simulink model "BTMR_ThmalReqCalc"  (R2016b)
settings: Solver=FixedStepDiscrete  StartTime=0.0  StopTime=10.0  FixedStep=0.1  RelTol=1e-3  EnableMultiTasking=on
undefined symbols (not defined in the file or in its folder): BMS_cntThmStbNum_C, BTMR_cntThmalReqVal_C, BTMR_flgCoolPwrCal_C, BTMR_pChrgClntPwrLv1_C, BTMR_pChrgClntPwrLv2_C, BTMR_pChrgClntPwrLv3_C, BTMR_pChrgClntPwrLv4_C, BTMR_pChrgClntPwrLv5_C, BTMR_pChrgClntPwrLv6_C, BTMR_pCoolPwrVal_C, BTMR_pHtgACPwrReq_C, BTMR_pHtgDCPwrReq_C, BTMR_pHtgDrvPwrReq_C, BTMR_pHtgsStage1_CUR, BTMR_pHtgsStage2_CUR, BTMR_pNormClntPwrLv1_C, BTMR_pNormClntPwrLv2_C, BTMR_pNormClntPwrLv3_C, BTMR_r861BrsDrvSoc_C, BTMR_r861HtgDrvSoc_C, BTMR_r891BrsDrvSoc_C, BTMR_r891HtgDrvSoc_C, BTMR_rCoolClbFlg_C, BTMR_rFlashClbFlg_C, BTMR_rHeatClbFlg_C, BTMR_t861BrsDiffLv0Temp_C, BTMR_t861BrsDiffLv1Temp_C, BTMR_t861CoolChrgAces2Temp_C, BTMR_t861CoolChrgAces3Temp_C, BTMR_t861CoolChrgAcesTemp_C, BTMR_t861CoolChrgDiffDebTemp_C, BTMR_t861CoolChrgEndDiffTemp_C, BTMR_t861CoolChrgExitLv2Temp_C, BTMR_t861CoolChrgExitLv3Temp_C, BTMR_t861CoolChrgExitTemp_C, BTMR_t861CoolChrgIntLv0Temp_C, BTMR_t861CoolChrgIntLv1Temp_C, BTMR_t861CoolChrgIntLv2Temp_C, BTMR_t861CoolChrgIntLv3Temp_C, BTMR_t861CoolChrgIntLv4Temp_C, BTMR_t861CoolChrgIntLv5Temp_C, BTMR_t861CoolDCDebTemp_C, BTMR_t861CoolNormAcesTemp_C, BTMR_t861CoolNormDiffDebTemp_C, BTMR_t861CoolNormEndDiffTemp_C, BTMR_t861CoolNormExitLv2Temp_C, BTMR_t861CoolNormExitLv3Temp_C, BTMR_t861CoolNormExitTemp_C, BTMR_t861CoolNormIntLv0Temp_C, BTMR_t861CoolNormIntLv1Temp_C, BTMR_t861CoolNormLv2Temp_C, BTMR_t861CoolNormLv3Temp_C, BTMR_t861HtgACDiffDebTemp_C, BTMR_t861HtgACEndDiffTemp_C, BTMR_t861HtgACStartHiTemp_C, BTMR_t861HtgACStartLoTemp_C, BTMR_t861HtgACStopTemp_C, BTMR_t861HtgDCDiffDebTemp_C, BTMR_t861HtgDCEndDiffTemp_C, BTMR_t861HtgDCIntLv0Temp_C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
libraries: AIWAYS_Powertrain_BMS_lib x78, simulink x9
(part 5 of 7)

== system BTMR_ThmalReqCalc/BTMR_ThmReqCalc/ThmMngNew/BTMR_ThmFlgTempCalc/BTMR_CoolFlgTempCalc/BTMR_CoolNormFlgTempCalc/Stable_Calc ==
  source_Uint : Inport
  cntStable : Inport  Port=2
  Chart : Stateflow chart  TreatAsAtomicUnit=on
  Delay1 : Delay  DelayLength=1  InitialCondition=0
  Detect Change : simulink/Logic and Bit Operations/Detect Change  vinit=0  OutDataTypeStr=boolean
  Switch : Switch  Criteria=u2 ~= 0
  stableOut : Outport
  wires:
  source_Uint/1 -> Detect Change/1, Switch/3
  Switch/1 -> stableOut/1, Delay1/1
  Delay1/1 -> Switch/1
  Chart/1(flg_out) -> Switch/2
  cntStable/1 -> Chart/2(cntStable)
  Detect Change/1 -> Chart/1(trigger_in)

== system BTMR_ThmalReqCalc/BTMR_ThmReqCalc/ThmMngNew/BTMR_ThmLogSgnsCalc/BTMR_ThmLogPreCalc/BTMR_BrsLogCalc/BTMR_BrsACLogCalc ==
  BTMR_flgBMSStsSgns : Inport
  BTMR_flgBrsEnSgns : Inport  Port=2
  BTMR_flgBrsIntSgns : Inport  Port=3
  Bus Creator : BusCreator  Inputs=3
  Bus Selector : BusSelector  OutputSignals=BTMR_flgBMSAChrg
  Bus Selector2 : BusSelector  OutputSignals=BTMR_flgBrsEna2Temp
  Bus Selector3 : BusSelector  OutputSignals=BTMR_flgBrsIntEna2Temp
  Logical Operator1 : Logic  Operator=NOT  AllPortsSameDT=off  OutDataTypeStr=boolean
  Logical Operator{2..4,6} (4 alike) : Logic  AllPortsSameDT=off  OutDataTypeStr=boolean
  Logical Operator5 : Logic  Operator=NOT  AllPortsSameDT=off  OutDataTypeStr=boolean
  BTMR_flgBrsACLogSgns : Outport
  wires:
  Bus Selector3/1 -> Logical Operator5/1, Logical Operator3/2  "<BTMR_flgBrsIntEna2Temp>"
  Logical Operator6/1 -> Logical Operator3/1, Logical Operator4/1  "BTMR_flgBrsEna2"
  Logical Operator2/1 -> Bus Creator/2  "BTMR_flgBrsACOut"
  Logical Operator1/1 -> Logical Operator2/2
  Bus Selector/1 -> Logical Operator2/1, Logical Operator6/1  "<BTMR_flgBMSAChrg>"
  BTMR_flgBrsEnSgns/1 -> Bus Selector2/1
  BTMR_flgBrsIntSgns/1 -> Bus Selector3/1
  BTMR_flgBMSStsSgns/1 -> Bus Selector/1
  Logical Operator4/1 -> Bus Creator/3  "BTMR_flgBrsACout2"
  Bus Selector2/1 -> Logical Operator1/1, Logical Operator6/2  "<BTMR_flgBrsEna2Temp>"
  Logical Operator3/1 -> Bus Creator/1  "BTMR_flgBrsIntEna2"
  Logical Operator5/1 -> Logical Operator4/2
  Bus Creator/1 -> BTMR_flgBrsACLogSgns/1  "BTMR_flgBrsACLogSgns"

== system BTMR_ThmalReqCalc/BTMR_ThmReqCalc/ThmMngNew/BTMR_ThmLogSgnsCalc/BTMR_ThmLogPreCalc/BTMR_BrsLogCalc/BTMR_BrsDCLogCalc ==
  BTMR_flgBMSStsSgns : Inport
  BTMR_flgBrsEnSgns : Inport  Port=2
  BTMR_flgBrsIntSgns : Inport  Port=3
  Bus Creator : BusCreator  Inputs=3
  Bus Selector : BusSelector  OutputSignals=BTMR_flgBMSDChrg
  Bus Selector2 : BusSelector  OutputSignals=BTMR_flgBrsEna1Temp
  Bus Selector3 : BusSelector  OutputSignals=BTMR_flgBrsIntEna1Temp
  Logical Operator1 : Logic  Operator=NOT  AllPortsSameDT=off  OutDataTypeStr=boolean
  Logical Operator{2..4,6} (4 alike) : Logic  AllPortsSameDT=off  OutDataTypeStr=boolean
  Logical Operator5 : Logic  Operator=NOT  AllPortsSameDT=off  OutDataTypeStr=boolean
  BTMR_flgBrsDCLogSgns : Outport
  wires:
  Bus Creator/1 -> BTMR_flgBrsDCLogSgns/1  "BTMR_flgBrsDCLogSgns"
  Logical Operator5/1 -> Logical Operator4/2
  Logical Operator3/1 -> Bus Creator/1  "BTMR_flgBrsIntEna1"
  Bus Selector2/1 -> Logical Operator6/2, Logical Operator1/1  "<BTMR_flgBrsEna1Temp>"
  Logical Operator4/1 -> Bus Creator/3  "BTMR_flgBrsDCout2"
  BTMR_flgBMSStsSgns/1 -> Bus Selector/1
  BTMR_flgBrsIntSgns/1 -> Bus Selector3/1
  BTMR_flgBrsEnSgns/1 -> Bus Selector2/1
  Bus Selector/1 -> Logical Operator6/1, Logical Operator2/1  "<BTMR_flgBMSDChrg>"
  Logical Operator1/1 -> Logical Operator2/2
  Logical Operator2/1 -> Bus Creator/2  "BTMR_flgBrsDCOut"
  Logical Operator6/1 -> Logical Operator3/1, Logical Operator4/1  "BTMR_flgBrsEna1"
  Bus Selector3/1 -> Logical Operator3/2, Logical Operator5/1  "<BTMR_flgBrsIntEna1Temp>"

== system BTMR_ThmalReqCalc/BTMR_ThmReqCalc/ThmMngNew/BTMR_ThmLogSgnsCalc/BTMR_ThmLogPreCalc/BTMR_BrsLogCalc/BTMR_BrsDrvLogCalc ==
  BTMR_flgBMSStsSgns : Inport
  BTMR_flgBrsEnSgns : Inport  Port=2
  BTMR_flgBrsIntSgns : Inport  Port=3
  BTMR_flgSOCSgns : Inport  Port=4
  Bus Creator : BusCreator  Inputs=4
  Bus Selector : BusSelector  OutputSignals=BTMR_flgBMSDrv
  Bus Selector1 : BusSelector  OutputSignals=BTMR_flgBrsDrvSOC
  Bus Selector2 : BusSelector  OutputSignals=BTMR_flgBrsEna3Temp
  Bus Selector3 : BusSelector  OutputSignals=BTMR_flgBrsIntEna3Temp
  Logical Operator1 : Logic  Operator=NOT  AllPortsSameDT=off  OutDataTypeStr=boolean
  Logical Operator{2..4,6..7,9} (6 alike) : Logic  AllPortsSameDT=off  OutDataTypeStr=boolean
  Logical Operator5 : Logic  Operator=NOT  AllPortsSameDT=off  OutDataTypeStr=boolean
  Logical Operator8 : Logic  Operator=NOT  AllPortsSameDT=off  OutDataTypeStr=boolean
  BTMR_flgBrsDrvLogSgns : Outport
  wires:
  Bus Creator/1 -> BTMR_flgBrsDrvLogSgns/1  "BTMR_flgBrsDrvLogSgns"
  Logical Operator5/1 -> Logical Operator4/2
  Logical Operator7/1 -> Bus Creator/1  "BTMR_flgBrsIntEna3"
  Bus Selector2/1 -> Logical Operator1/1, Logical Operator6/2  "<BTMR_flgBrsEna3Temp>"
  Logical Operator9/1 -> Bus Creator/3  "BTMR_flgBrsDrvOut2"
  BTMR_flgBMSStsSgns/1 -> Bus Selector/1
  BTMR_flgBrsIntSgns/1 -> Bus Selector3/1
  BTMR_flgBrsEnSgns/1 -> Bus Selector2/1
  Bus Selector/1 -> Logical Operator6/1, Logical Operator2/1  "<BTMR_flgBMSDrv>"
  Logical Operator1/1 -> Logical Operator2/2
  Logical Operator6/1 -> Logical Operator9/1, Logical Operator3/1  "BTMR_flgBrsEna3"
  Bus Selector3/1 -> Logical Operator5/1, Logical Operator7/2  "<BTMR_flgBrsIntEna3Temp>"
  BTMR_flgSOCSgns/1 -> Bus Selector1/1
  Bus Selector1/1 -> Logical Operator3/2, Logical Operator8/1  "<BTMR_flgBrsDrvSOC>"
  Logical Operator3/1 -> Logical Operator4/1, Logical Operator7/1  "BTMR_flgBrsSOCEna3"
  Logical Operator2/1 -> Bus Creator/2  "BTMR_flgBrsDrvOut"
  Logical Operator8/1 -> Logical Operator9/2
  Logical Operator4/1 -> Bus Creator/4  "BTMR_flgBrsDrvOut3"

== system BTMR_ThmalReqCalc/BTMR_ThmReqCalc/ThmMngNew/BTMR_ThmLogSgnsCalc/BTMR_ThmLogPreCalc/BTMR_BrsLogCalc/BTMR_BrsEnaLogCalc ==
  BTMR_flgBrsDCLogSgns : Inport
  BTMR_flgBrsACLogSgns : Inport  Port=2
  BTMR_flgBrsDrvLogSgns : Inport  Port=3
  BTMR_flgBrsTempSgns : Inport  Port=4
  BTMR_BrsEnaCalc : Subsystem
  Bus Creator : BusCreator  Inputs=3
  Bus Creator2 : BusCreator  Inputs=2
  Bus Selector : BusSelector  OutputSignals=BTMR_flgBrsInTempSgns,BTMR_flgBrsCellIntTempSgn
  Bus Selector2 : BusSelector  OutputSignals=BTMR_flgBrsStartTemp
  Logical Operator1 : Logic  Operator=NOT  AllPortsSameDT=off  OutDataTypeStr=boolean
  Logical Operator2 : Logic  AllPortsSameDT=off  OutDataTypeStr=boolean
  Logical Operator3 : Logic  AllPortsSameDT=off  OutDataTypeStr=boolean
  BTMR_flgBrsEnaLogSgns : Outport
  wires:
  BTMR_flgBrsDCLogSgns/1 -> Bus Creator/1
  BTMR_flgBrsACLogSgns/1 -> Bus Creator/2
  BTMR_flgBrsDrvLogSgns/1 -> Bus Creator/3
  Bus Creator/1 -> BTMR_BrsEnaCalc/1(BTMR_flgBrsInLogSgns)  "BTMR_flgBrsInLogSgns"
  Bus Selector/1 -> Bus Selector2/1  "<BTMR_flgBrsInTempSgns>"
  Bus Selector2/1 -> Logical Operator1/1  "<BTMR_flgBrsStartTemp>"
  BTMR_BrsEnaCalc/1(BTMR_flgBrsEna) -> Logical Operator3/1, Logical Operator2/1
  Logical Operator1/1 -> Logical Operator3/2
  Logical Operator3/1 -> Bus Creator2/2  "BTMR_flgBrsOut"
  BTMR_flgBrsTempSgns/1 -> Bus Selector/1
  Bus Creator2/1 -> BTMR_flgBrsEnaLogSgns/1  "BTMR_flgBrsEnaLogSgns"
  Logical Operator2/1 -> Bus Creator2/1  "BTMR_flgBrsEna"
  Bus Selector/2 -> Logical Operator2/2  "<BTMR_flgBrsCellIntTempSgn>"

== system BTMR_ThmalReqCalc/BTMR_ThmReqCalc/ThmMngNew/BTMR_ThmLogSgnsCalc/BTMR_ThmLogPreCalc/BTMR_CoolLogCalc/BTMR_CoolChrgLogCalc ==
  BTMR_flgHtgLogSgns : Inport
  BTMR_flgThmEnaTempSgns : Inport  Port=2
  Bus Creator : BusCreator  Inputs=2
  Bus Selector : BusSelector  OutputSignals=BTMR_flgHtgDCLogSgns
  Bus Selector1 : BusSelector  OutputSignals=BTMR_flgHtgDCOut
  Bus Selector2 : BusSelector  OutputSignals=BTMR_CoolChrgEnaTemp
  Logical Operator1 : Logic  Operator=NOT  AllPortsSameDT=off  OutDataTypeStr=boolean
  Logical Operator2 : Logic  AllPortsSameDT=off  OutDataTypeStr=boolean
  Logical Operator3 : Logic  AllPortsSameDT=off  OutDataTypeStr=boolean
  BTMR_flgCoolChrgLogSgns : Outport
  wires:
  Bus Creator/1 -> BTMR_flgCoolChrgLogSgns/1  "BTMR_flgCoolChrgLogSgns"
  BTMR_flgThmEnaTempSgns/1 -> Bus Selector2/1
  Bus Selector1/1 -> Logical Operator3/1, Logical Operator2/1  "<BTMR_flgHtgDCOut>"
  Bus Selector2/1 -> Logical Operator1/1, Logical Operator3/2  "<BTMR_CoolChrgEnaTemp>"
  Logical Operator1/1 -> Logical Operator2/2
  Logical Operator3/1 -> Bus Creator/1  "BTMR_flgCoolChrgEna"
  Logical Operator2/1 -> Bus Creator/2  "BTMR_flgCoolChrgOut"
  Bus Selector/1 -> Bus Selector1/1  "<BTMR_flgHtgDCLogSgns>"
  BTMR_flgHtgLogSgns/1 -> Bus Selector/1

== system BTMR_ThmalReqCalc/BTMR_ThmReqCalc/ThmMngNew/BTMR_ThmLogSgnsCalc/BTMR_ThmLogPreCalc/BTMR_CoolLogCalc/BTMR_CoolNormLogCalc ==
  BTMR_flgHtgLogSgns : Inport
  BTMR_flgThmEnaTempSgns : Inport  Port=2
  Bus Creator : BusCreator  Inputs=2
  Bus Selector : BusSelector  OutputSignals=BTMR_flgHtgACLogSgns,BTMR_flgHtgDrvLogSgns
  Bus Selector1 : BusSelector  OutputSignals=BTMR_flgHtgACOut
  Bus Selector2 : BusSelector  OutputSignals=BTMR_CoolNormEnaTemp
  Bus Selector3 : BusSelector  OutputSignals=BTMR_flgHtgDrvOut
  Logical Operator1 : Logic  Operator=NOT  AllPortsSameDT=off  OutDataTypeStr=boolean
  Logical Operator2 : Logic  AllPortsSameDT=off  OutDataTypeStr=boolean
  Logical Operator3 : Logic  AllPortsSameDT=off  OutDataTypeStr=boolean
  Logical Operator4 : Logic  Operator=OR  AllPortsSameDT=off  OutDataTypeStr=boolean
  BTMR_flgCoolNormLogSgns : Outport
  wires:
  BTMR_flgHtgLogSgns/1 -> Bus Selector/1
  Bus Selector/1 -> Bus Selector1/1  "<BTMR_flgHtgACLogSgns>"
  Logical Operator2/1 -> Bus Creator/2  "BTMR_flgCoolNormOut"
  Logical Operator3/1 -> Bus Creator/1  "BTMR_flgCoolNormEna"
  Logical Operator1/1 -> Logical Operator2/2
  Bus Selector2/1 -> Logical Operator3/2, Logical Operator1/1  "<BTMR_CoolNormEnaTemp>"
  Logical Operator4/1 -> Logical Operator2/1, Logical Operator3/1
  BTMR_flgThmEnaTempSgns/1 -> Bus Selector2/1
  Bus Creator/1 -> BTMR_flgCoolNormLogSgns/1  "BTMR_flgCoolNormLogSgns"
  Bus Selector/2 -> Bus Selector3/1  "<BTMR_flgHtgDrvLogSgns>"
  Bus Selector1/1 -> Logical Operator4/1  "<BTMR_flgHtgACOut>"
  Bus Selector3/1 -> Logical Operator4/2  "<BTMR_flgHtgDrvOut>"

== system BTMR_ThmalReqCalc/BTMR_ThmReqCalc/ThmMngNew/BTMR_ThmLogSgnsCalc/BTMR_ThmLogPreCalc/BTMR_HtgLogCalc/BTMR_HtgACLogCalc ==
  BTMR_flgBrsLogSgns : Inport
  BTMR_flgThmEnaTempSgns : Inport  Port=2
  Bus Creator : BusCreator  Inputs=2
  Bus Selector : BusSelector  OutputSignals=BTMR_flgBrsACLogSgns
  Bus Selector1 : BusSelector  OutputSignals=BTMR_flgBrsACOut
  Bus Selector2 : BusSelector  OutputSignals=BTMR_HtgACEnaTemp
  Logical Operator1 : Logic  Operator=NOT  AllPortsSameDT=off  OutDataTypeStr=boolean
  Logical Operator2 : Logic  AllPortsSameDT=off  OutDataTypeStr=boolean
  Logical Operator3 : Logic  AllPortsSameDT=off  OutDataTypeStr=boolean
  BTMR_flgHtgACLogSgns : Outport
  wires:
  Bus Creator/1 -> BTMR_flgHtgACLogSgns/1  "BTMR_flgHtgACLogSgns"
  BTMR_flgThmEnaTempSgns/1 -> Bus Selector2/1
  Bus Selector1/1 -> Logical Operator3/1, Logical Operator2/1  "<BTMR_flgBrsACOut>"
  Bus Selector2/1 -> Logical Operator1/1, Logical Operator3/2  "<BTMR_HtgACEnaTemp>"
  Logical Operator1/1 -> Logical Operator2/2
  Logical Operator3/1 -> Bus Creator/1  "BTMR_flgHtgACEna"
  Logical Operator2/1 -> Bus Creator/2  "BTMR_flgHtgACOut"
  Bus Selector/1 -> Bus Selector1/1  "<BTMR_flgBrsACLogSgns>"
  BTMR_flgBrsLogSgns/1 -> Bus Selector/1

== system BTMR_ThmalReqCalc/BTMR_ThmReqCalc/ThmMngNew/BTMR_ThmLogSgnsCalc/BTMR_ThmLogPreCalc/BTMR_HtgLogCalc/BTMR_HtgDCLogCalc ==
  BTMR_flgBrsLogSgns : Inport
  BTMR_flgThmEnaTempSgns : Inport  Port=2
  Bus Creator : BusCreator  Inputs=2
  Bus Selector : BusSelector  OutputSignals=BTMR_flgBrsDCLogSgns
  Bus Selector1 : BusSelector  OutputSignals=BTMR_flgBrsDCOut
  Bus Selector2 : BusSelector  OutputSignals=BTMR_HtgDCEnaTemp
  Logical Operator1 : Logic  Operator=NOT  AllPortsSameDT=off  OutDataTypeStr=boolean
  Logical Operator2 : Logic  AllPortsSameDT=off  OutDataTypeStr=boolean
  Logical Operator3 : Logic  AllPortsSameDT=off  OutDataTypeStr=boolean
  BTMR_flgHtgDCLogSgns : Outport
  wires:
  BTMR_flgBrsLogSgns/1 -> Bus Selector/1
  Bus Selector/1 -> Bus Selector1/1  "<BTMR_flgBrsDCLogSgns>"
  Logical Operator2/1 -> Bus Creator/2  "BTMR_flgHtgDCOut"
  Logical Operator3/1 -> Bus Creator/1  "BTMR_flgHtgDCEna"
  Logical Operator1/1 -> Logical Operator2/2
  Bus Selector2/1 -> Logical Operator3/2, Logical Operator1/1  "<BTMR_HtgDCEnaTemp>"
  Bus Selector1/1 -> Logical Operator2/1, Logical Operator3/1  "<BTMR_flgBrsDCOut>"
  BTMR_flgThmEnaTempSgns/1 -> Bus Selector2/1
  Bus Creator/1 -> BTMR_flgHtgDCLogSgns/1  "BTMR_flgHtgDCLogSgns"

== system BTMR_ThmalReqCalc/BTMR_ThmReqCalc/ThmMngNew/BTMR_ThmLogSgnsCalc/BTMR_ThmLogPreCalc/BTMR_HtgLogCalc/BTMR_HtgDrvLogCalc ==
  BTMR_flgBrsLogSgns : Inport
  BTMR_flgThmEnaTempSgns : Inport  Port=2
  Bus Creator : BusCreator  Inputs=2
  Bus Selector : BusSelector  OutputSignals=BTMR_flgBrsDrvLogSgns
  Bus Selector1 : BusSelector  OutputSignals=BTMR_flgBrsDrvOut
  Bus Selector2 : BusSelector  OutputSignals=BTMR_HtgDrvEnaTemp
  Logical Operator1 : Logic  Operator=NOT  AllPortsSameDT=off  OutDataTypeStr=boolean
  Logical Operator2 : Logic  AllPortsSameDT=off  OutDataTypeStr=boolean
  Logical Operator3 : Logic  AllPortsSameDT=off  OutDataTypeStr=boolean
  BTMR_flgHtgDrvLogSgns : Outport
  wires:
  BTMR_flgBrsLogSgns/1 -> Bus Selector/1
  Bus Selector/1 -> Bus Selector1/1  "<BTMR_flgBrsDrvLogSgns>"
  Logical Operator2/1 -> Bus Creator/2  "BTMR_flgHtgDrvOut"
  Logical Operator1/1 -> Logical Operator2/2
  Bus Selector2/1 -> Logical Operator3/2, Logical Operator1/1  "<BTMR_HtgDrvEnaTemp>"
  Bus Selector1/1 -> Logical Operator2/1, Logical Operator3/1  "<BTMR_flgBrsDrvOut>"
  BTMR_flgThmEnaTempSgns/1 -> Bus Selector2/1
  Bus Creator/1 -> BTMR_flgHtgDrvLogSgns/1  "BTMR_flgHtgDrvLogSgns"
  Logical Operator3/1 -> Bus Creator/1  "BTMR_flgHtgDrvEna"

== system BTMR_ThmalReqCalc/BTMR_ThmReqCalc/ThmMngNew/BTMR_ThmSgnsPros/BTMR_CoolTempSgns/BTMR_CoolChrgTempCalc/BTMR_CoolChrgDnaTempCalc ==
  BSPR_tCellTempMax : Inport
  BMSDebounceStartZero : AIWAYS_Powertrain_BMS_lib/Debounce & Delay/BMSDebounceStartZero
  Constant1 : Constant  Value=BTMR_tiTempBase_C
  Constant14 : Constant  Value=BTMR_t891CoolChrgExitTemp_C
  Constant2 : Constant  Value=BTMR_tiTempDebs_C
  Relational Operator20 : RelationalOperator  Operator=<=  OutDataTypeStr=boolean  RndMeth=Simplest
  BTMR_flgCoolChrgDnaTemp : Outport
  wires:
  Relational Operator20/1 -> BMSDebounceStartZero/1
  BMSDebounceStartZero/1 -> BTMR_flgCoolChrgDnaTemp/1
  BSPR_tCellTempMax/1 -> Relational Operator20/1
  Constant14/1 -> Relational Operator20/2
  Constant2/1 -> BMSDebounceStartZero/4, BMSDebounceStartZero/2
  Constant1/1 -> BMSDebounceStartZero/5, BMSDebounceStartZero/3

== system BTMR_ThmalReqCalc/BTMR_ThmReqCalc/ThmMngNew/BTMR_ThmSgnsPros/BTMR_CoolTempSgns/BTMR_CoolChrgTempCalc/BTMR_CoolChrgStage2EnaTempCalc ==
  BSPR_tCellTempMax : Inport
  BMSDebounceStartZero : AIWAYS_Powertrain_BMS_lib/Debounce & Delay/BMSDebounceStartZero
  Constant1 : Constant  Value=BTMR_tiTempBase_C
  Constant15 : Constant  Value=BTMR_t891CoolChrgAces2Temp_C
  Constant2 : Constant  Value=BTMR_tiTempDebs_C
  Relational Operator20 : RelationalOperator  OutDataTypeStr=boolean  RndMeth=Simplest
  BTMR_flgCoolChrgStage2EnaTemp : Outport
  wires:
  Relational Operator20/1 -> BMSDebounceStartZero/1
  BMSDebounceStartZero/1 -> BTMR_flgCoolChrgStage2EnaTemp/1
  BSPR_tCellTempMax/1 -> Relational Operator20/1
  Constant15/1 -> Relational Operator20/2
  Constant2/1 -> BMSDebounceStartZero/4, BMSDebounceStartZero/2
  Constant1/1 -> BMSDebounceStartZero/5, BMSDebounceStartZero/3

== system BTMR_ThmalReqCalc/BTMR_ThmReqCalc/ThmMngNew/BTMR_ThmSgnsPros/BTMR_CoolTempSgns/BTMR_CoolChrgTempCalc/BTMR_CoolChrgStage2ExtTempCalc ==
  BSPR_tCellTempMax : Inport
  BMSDebounceStartZero : AIWAYS_Powertrain_BMS_lib/Debounce & Delay/BMSDebounceStartZero
  Constant1 : Constant  Value=BTMR_tiTempBase_C
  Constant13 : Constant  Value=BTMR_t891CoolChrgExitLv2Temp_C
  Constant2 : Constant  Value=BTMR_tiTempDebs_C
  Relational Operator20 : RelationalOperator  Operator=<=  OutDataTypeStr=boolean  RndMeth=Simplest
  BTMR_flgCoolChrgStage2ExtTemp : Outport
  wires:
  Constant13/1 -> Relational Operator20/2
  BSPR_tCellTempMax/1 -> Relational Operator20/1
  BMSDebounceStartZero/1 -> BTMR_flgCoolChrgStage2ExtTemp/1
  Relational Operator20/1 -> BMSDebounceStartZero/1
  Constant2/1 -> BMSDebounceStartZero/4, BMSDebounceStartZero/2
  Constant1/1 -> BMSDebounceStartZero/5, BMSDebounceStartZero/3

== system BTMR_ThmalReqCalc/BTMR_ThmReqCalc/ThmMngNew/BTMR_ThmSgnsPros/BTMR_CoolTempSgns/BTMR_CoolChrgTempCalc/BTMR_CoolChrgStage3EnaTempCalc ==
  BSPR_tCellTempMax : Inport
  BMSDebounceStartZero : AIWAYS_Powertrain_BMS_lib/Debounce & Delay/BMSDebounceStartZero
  Constant1 : Constant  Value=BTMR_tiTempBase_C
  Constant13 : Constant  Value=BTMR_t891CoolChrgAces3Temp_C
  Constant2 : Constant  Value=BTMR_tiTempDebs_C
  Relational Operator20 : RelationalOperator  OutDataTypeStr=boolean  RndMeth=Simplest
  BTMR_flgCoolChrgStage3EnaTemp : Outport
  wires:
  Constant13/1 -> Relational Operator20/2
  BSPR_tCellTempMax/1 -> Relational Operator20/1
  BMSDebounceStartZero/1 -> BTMR_flgCoolChrgStage3EnaTemp/1
  Relational Operator20/1 -> BMSDebounceStartZero/1
  Constant2/1 -> BMSDebounceStartZero/4, BMSDebounceStartZero/2
  Constant1/1 -> BMSDebounceStartZero/5, BMSDebounceStartZero/3

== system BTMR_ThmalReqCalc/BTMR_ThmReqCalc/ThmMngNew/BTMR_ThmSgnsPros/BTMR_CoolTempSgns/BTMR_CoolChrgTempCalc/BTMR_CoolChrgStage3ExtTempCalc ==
  BSPR_tCellTempMax : Inport
  BMSDebounceStartZero : AIWAYS_Powertrain_BMS_lib/Debounce & Delay/BMSDebounceStartZero
  Constant1 : Constant  Value=BTMR_tiTempBase_C
  Constant13 : Constant  Value=BTMR_t891CoolChrgExitLv3Temp_C
  Constant2 : Constant  Value=BTMR_tiTempDebs_C
  Relational Operator20 : RelationalOperator  Operator=<=  OutDataTypeStr=boolean  RndMeth=Simplest
  BTMR_flgCoolChrgStage3ExtTemp : Outport
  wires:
  Relational Operator20/1 -> BMSDebounceStartZero/1
  BSPR_tCellTempMax/1 -> Relational Operator20/1
  Constant13/1 -> Relational Operator20/2
  BMSDebounceStartZero/1 -> BTMR_flgCoolChrgStage3ExtTemp/1
  Constant2/1 -> BMSDebounceStartZero/4, BMSDebounceStartZero/2
  Constant1/1 -> BMSDebounceStartZero/5, BMSDebounceStartZero/3

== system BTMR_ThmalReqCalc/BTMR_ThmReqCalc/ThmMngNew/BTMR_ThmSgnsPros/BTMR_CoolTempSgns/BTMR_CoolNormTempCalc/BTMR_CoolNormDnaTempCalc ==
  BSPR_tCellTempMax : Inport
  BMSDebounceStartZero : AIWAYS_Powertrain_BMS_lib/Debounce & Delay/BMSDebounceStartZero
  Constant1 : Constant  Value=BTMR_tiTempBase_C
  Constant13 : Constant  Value=BTMR_t891CoolNormExitTemp_C
  Constant2 : Constant  Value=BTMR_tiTempDebs_C
  Relational Operator20 : RelationalOperator  Operator=<=  OutDataTypeStr=boolean  RndMeth=Simplest
  BTMR_flgCoolNormDnaTemp : Outport
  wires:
  BSPR_tCellTempMax/1 -> Relational Operator20/1
  Constant13/1 -> Relational Operator20/2
  BMSDebounceStartZero/1 -> BTMR_flgCoolNormDnaTemp/1
  Relational Operator20/1 -> BMSDebounceStartZero/1
  Constant2/1 -> BMSDebounceStartZero/4, BMSDebounceStartZero/2
  Constant1/1 -> BMSDebounceStartZero/5, BMSDebounceStartZero/3

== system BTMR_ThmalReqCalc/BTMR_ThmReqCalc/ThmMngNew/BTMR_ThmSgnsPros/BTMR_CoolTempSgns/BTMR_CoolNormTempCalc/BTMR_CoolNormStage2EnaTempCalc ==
  BSPR_tCellTempMax : Inport
  BMSDebounceStartZero : AIWAYS_Powertrain_BMS_lib/Debounce & Delay/BMSDebounceStartZero
  Constant1 : Constant  Value=BTMR_t891CoolNormLv2Temp_C
  Constant2 : Constant  Value=BTMR_tiTempBase_C
  Constant3 : Constant  Value=BTMR_tiTempDebs_C
  Relational Operator20 : RelationalOperator  OutDataTypeStr=boolean  RndMeth=Simplest
  BTMR_flgCoolNormStage2EnaTemp : Outport
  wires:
  BSPR_tCellTempMax/1 -> Relational Operator20/1
  Constant1/1 -> Relational Operator20/2
  BMSDebounceStartZero/1 -> BTMR_flgCoolNormStage2EnaTemp/1
  Relational Operator20/1 -> BMSDebounceStartZero/1
  Constant3/1 -> BMSDebounceStartZero/4, BMSDebounceStartZero/2
  Constant2/1 -> BMSDebounceStartZero/5, BMSDebounceStartZero/3

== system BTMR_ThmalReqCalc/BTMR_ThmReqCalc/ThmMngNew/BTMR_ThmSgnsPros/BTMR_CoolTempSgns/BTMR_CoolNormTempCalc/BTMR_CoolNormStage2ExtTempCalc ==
  BSPR_tCellTempMax : Inport
  BMSDebounceStartZero : AIWAYS_Powertrain_BMS_lib/Debounce & Delay/BMSDebounceStartZero
  Constant1 : Constant  Value=BTMR_tiTempBase_C
  Constant13 : Constant  Value=BTMR_t891CoolNormExitLv2Temp_C
  Constant2 : Constant  Value=BTMR_tiTempDebs_C
  Relational Operator20 : RelationalOperator  Operator=<=  OutDataTypeStr=boolean  RndMeth=Simplest
  BTMR_flgCoolNormStage2ExtTemp : Outport
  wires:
  Relational Operator20/1 -> BMSDebounceStartZero/1
  BMSDebounceStartZero/1 -> BTMR_flgCoolNormStage2ExtTemp/1
  Constant13/1 -> Relational Operator20/2
  BSPR_tCellTempMax/1 -> Relational Operator20/1
  Constant2/1 -> BMSDebounceStartZero/4, BMSDebounceStartZero/2
  Constant1/1 -> BMSDebounceStartZero/5, BMSDebounceStartZero/3

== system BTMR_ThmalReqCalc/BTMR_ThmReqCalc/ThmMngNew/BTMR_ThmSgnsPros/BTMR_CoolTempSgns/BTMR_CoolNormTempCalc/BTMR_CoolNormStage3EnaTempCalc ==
  BSPR_tCellTempMax : Inport
  BMSDebounceStartZero : AIWAYS_Powertrain_BMS_lib/Debounce & Delay/BMSDebounceStartZero
  Constant1 : Constant  Value=BTMR_t891CoolNormLv3Temp_C
  Constant2 : Constant  Value=BTMR_tiTempBase_C
  Constant3 : Constant  Value=BTMR_tiTempDebs_C
  Relational Operator20 : RelationalOperator  OutDataTypeStr=boolean  RndMeth=Simplest
  BTMR_flgCoolNormStage3EnaTemp : Outport
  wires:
  Relational Operator20/1 -> BMSDebounceStartZero/1
  BMSDebounceStartZero/1 -> BTMR_flgCoolNormStage3EnaTemp/1
  Constant1/1 -> Relational Operator20/2
  BSPR_tCellTempMax/1 -> Relational Operator20/1
  Constant3/1 -> BMSDebounceStartZero/4, BMSDebounceStartZero/2
  Constant2/1 -> BMSDebounceStartZero/5, BMSDebounceStartZero/3

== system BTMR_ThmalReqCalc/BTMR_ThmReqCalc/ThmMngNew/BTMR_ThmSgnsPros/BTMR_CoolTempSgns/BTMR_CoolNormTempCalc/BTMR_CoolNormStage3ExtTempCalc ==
  BSPR_tCellTempMax : Inport
  BMSDebounceStartZero : AIWAYS_Powertrain_BMS_lib/Debounce & Delay/BMSDebounceStartZero
  Constant1 : Constant  Value=BTMR_tiTempBase_C
  Constant13 : Constant  Value=BTMR_t891CoolNormExitLv3Temp_C
  Constant2 : Constant  Value=BTMR_tiTempDebs_C
  Relational Operator20 : RelationalOperator  Operator=<=  OutDataTypeStr=boolean  RndMeth=Simplest
  BTMR_flgCoolNormStage3ExtTemp : Outport
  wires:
  BSPR_tCellTempMax/1 -> Relational Operator20/1
  Constant13/1 -> Relational Operator20/2
  BMSDebounceStartZero/1 -> BTMR_flgCoolNormStage3ExtTemp/1
  Relational Operator20/1 -> BMSDebounceStartZero/1
  Constant2/1 -> BMSDebounceStartZero/4, BMSDebounceStartZero/2
  Constant1/1 -> BMSDebounceStartZero/5, BMSDebounceStartZero/3

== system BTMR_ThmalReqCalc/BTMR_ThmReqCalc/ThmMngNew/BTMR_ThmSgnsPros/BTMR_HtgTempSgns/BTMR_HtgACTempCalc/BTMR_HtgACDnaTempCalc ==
  BSPR_tCellTempMin : Inport
  BSPR_tCellTempMax : Inport  Port=2
  BMSDebounceStartZero : AIWAYS_Powertrain_BMS_lib/Debounce & Delay/BMSDebounceStartZero
  Constant1 : Constant  Value=BTMR_t891HtgACStopMxTemp_C
  Constant2 : Constant  Value=BTMR_tiTempBase_C
  Constant3 : Constant  Value=BTMR_tiTempDebs_C
  Constant8 : Constant  Value=BTMR_t891HtgACStopTemp_C
  Logical Operator4 : Logic  Operator=OR  AllPortsSameDT=off  OutDataTypeStr=boolean
  Relational Operator1 : RelationalOperator  OutDataTypeStr=boolean  RndMeth=Simplest
  Relational Operator18 : RelationalOperator  OutDataTypeStr=boolean  RndMeth=Simplest
  BTMR_flgHtgACDnaTemp : Outport
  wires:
  Constant8/1 -> Relational Operator18/2
  BMSDebounceStartZero/1 -> BTMR_flgHtgACDnaTemp/1
  BSPR_tCellTempMin/1 -> Relational Operator18/1
  Relational Operator18/1 -> Logical Operator4/1
  Logical Operator4/1 -> BMSDebounceStartZero/1
  Constant1/1 -> Relational Operator1/2
  BSPR_tCellTempMax/1 -> Relational Operator1/1
  Relational Operator1/1 -> Logical Operator4/2
  Constant3/1 -> BMSDebounceStartZero/4, BMSDebounceStartZero/2
  Constant2/1 -> BMSDebounceStartZero/5, BMSDebounceStartZero/3

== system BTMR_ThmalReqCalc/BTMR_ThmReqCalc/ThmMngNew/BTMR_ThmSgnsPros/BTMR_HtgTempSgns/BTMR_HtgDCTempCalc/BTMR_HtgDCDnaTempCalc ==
  BSPR_tCellTempMin : Inport
  BSPR_tCellTempMax : Inport  Port=2
  BMSDebounceStartZero : AIWAYS_Powertrain_BMS_lib/Debounce & Delay/BMSDebounceStartZero
  Constant1 : Constant  Value=BTMR_tiTempBase_C
  Constant16 : Constant  Value=BTMR_t891HtgDCStopMinTemp_C
  Constant2 : Constant  Value=BTMR_tiTempDebs_C
  Constant23 : Constant  Value=BTMR_t891HtgDCStopMaxTemp_C
  Logical Operator4 : Logic  Operator=OR  AllPortsSameDT=off  OutDataTypeStr=boolean
  Relational Operator13 : RelationalOperator  OutDataTypeStr=boolean  RndMeth=Simplest
  Relational Operator18 : RelationalOperator  OutDataTypeStr=boolean  RndMeth=Simplest
  BTMR_flgHtgDCDnaTemp : Outport
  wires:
  BSPR_tCellTempMin/1 -> Relational Operator18/1
  Relational Operator18/1 -> Logical Operator4/1
  BMSDebounceStartZero/1 -> BTMR_flgHtgDCDnaTemp/1
  Constant16/1 -> Relational Operator18/2
  Relational Operator13/1 -> Logical Operator4/2
  Constant23/1 -> Relational Operator13/2
  BSPR_tCellTempMax/1 -> Relational Operator13/1
  Logical Operator4/1 -> BMSDebounceStartZero/1
  Constant2/1 -> BMSDebounceStartZero/4, BMSDebounceStartZero/2
  Constant1/1 -> BMSDebounceStartZero/5, BMSDebounceStartZero/3

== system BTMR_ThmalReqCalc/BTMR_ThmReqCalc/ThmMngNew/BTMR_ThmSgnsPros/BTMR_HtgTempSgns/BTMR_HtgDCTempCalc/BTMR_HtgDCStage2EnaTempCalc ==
  BSPR_tCellTempMin : Inport
  BSPR_tCellTempMax : Inport  Port=2
  BMSDebounceStartZero : AIWAYS_Powertrain_BMS_lib/Debounce & Delay/BMSDebounceStartZero
  Constant1 : Constant  Value=BTMR_tiTempBase_C
  Constant2 : Constant  Value=BTMR_tiTempDebs_C
  Constant23 : Constant  Value=BTMR_t891HtgDCStageMxTemp_C
  Constant24 : Constant  Value=BTMR_t891HtgDCStageMnTemp_C
  Logical Operator1 : Logic  Operator=NOT  AllPortsSameDT=off  OutDataTypeStr=boolean
  Logical Operator4 : Logic  AllPortsSameDT=off  OutDataTypeStr=boolean
  Relational Operator12 : RelationalOperator  Operator=<  OutDataTypeStr=boolean  RndMeth=Simplest
  Relational Operator13 : RelationalOperator  Operator=<  OutDataTypeStr=boolean  RndMeth=Simplest
  BTMR_flgHtgDCStage2EnaTemp : Outport
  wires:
  BSPR_tCellTempMin/1 -> Relational Operator12/1
  Logical Operator4/1 -> Logical Operator1/1
  Constant24/1 -> Relational Operator12/2
  Relational Operator13/1 -> Logical Operator4/2
  Constant23/1 -> Relational Operator13/2
  Relational Operator12/1 -> Logical Operator4/1
  BMSDebounceStartZero/1 -> BTMR_flgHtgDCStage2EnaTemp/1
  BSPR_tCellTempMax/1 -> Relational Operator13/1
  Logical Operator1/1 -> BMSDebounceStartZero/1
  Constant2/1 -> BMSDebounceStartZero/4, BMSDebounceStartZero/2
  Constant1/1 -> BMSDebounceStartZero/5, BMSDebounceStartZero/3

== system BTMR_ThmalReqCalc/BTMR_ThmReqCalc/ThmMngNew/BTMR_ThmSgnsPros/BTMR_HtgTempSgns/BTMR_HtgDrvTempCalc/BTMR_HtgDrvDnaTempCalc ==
  BSPR_tCellTempMin : Inport
  BSPR_tCellTempMax : Inport  Port=2
  BMSDebounceStartZero : AIWAYS_Powertrain_BMS_lib/Debounce & Delay/BMSDebounceStartZero
  Constant1 : Constant  Value=BTMR_t891HtgDrvStopMxTemp_C
  Constant2 : Constant  Value=BTMR_t891HtgDrvStopTemp_C
  Constant3 : Constant  Value=BTMR_tiTempBase_C
  Constant4 : Constant  Value=BTMR_tiTempDebs_C
  Logical Operator4 : Logic  Operator=OR  AllPortsSameDT=off  OutDataTypeStr=boolean
  Relational Operator1 : RelationalOperator  OutDataTypeStr=boolean  RndMeth=Simplest
  Relational Operator18 : RelationalOperator  OutDataTypeStr=boolean  RndMeth=Simplest
  BTMR_flgHtgDrvDnaTemp : Outport
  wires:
  BSPR_tCellTempMin/1 -> Relational Operator18/1
  BMSDebounceStartZero/1 -> BTMR_flgHtgDrvDnaTemp/1
  Constant2/1 -> Relational Operator18/2
  Relational Operator18/1 -> Logical Operator4/1
  Logical Operator4/1 -> BMSDebounceStartZero/1
  Constant1/1 -> Relational Operator1/2
  BSPR_tCellTempMax/1 -> Relational Operator1/1
  Relational Operator1/1 -> Logical Operator4/2
  Constant4/1 -> BMSDebounceStartZero/4, BMSDebounceStartZero/2
  Constant3/1 -> BMSDebounceStartZero/5, BMSDebounceStartZero/3

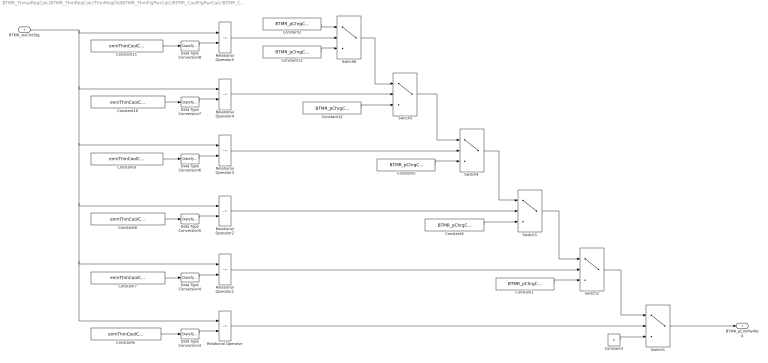
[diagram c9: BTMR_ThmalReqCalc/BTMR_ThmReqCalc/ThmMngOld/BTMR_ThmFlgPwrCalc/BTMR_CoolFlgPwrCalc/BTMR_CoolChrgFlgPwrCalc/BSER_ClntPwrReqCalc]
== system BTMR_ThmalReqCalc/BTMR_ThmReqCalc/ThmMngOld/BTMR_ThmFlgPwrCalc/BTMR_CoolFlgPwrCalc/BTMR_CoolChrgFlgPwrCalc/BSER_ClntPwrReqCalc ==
  BTMR_stsClntStg : Inport
  Constant1 : Constant  Value=BTMR_pChrgClntPwrLv1_C
  Constant10 : Constant  Value=enmThmCoolChrgStg_861.Stg_Lv2Res  OutDataTypeStr=Enum: enmThmCoolChrgStg_861
  Constant11 : Constant  Value=enmThmCoolChrgStg_861.Stg_Lv3Red  OutDataTypeStr=Enum: enmThmCoolChrgStg_861
  Constant12 : Constant  Value=BTMR_pChrgClntPwrLv4_C
  Constant13 : Constant  Value=BTMR_pChrgClntPwrLv5_C
  Constant2 : Constant  Value=BTMR_pChrgClntPwrLv6_C
  Constant3 : Constant  Value=0  OutDataTypeStr=single
  Constant4 : Constant  Value=BTMR_pChrgClntPwrLv2_C
  Constant5 : Constant  Value=BTMR_pChrgClntPwrLv3_C
  Constant6 : Constant  Value=enmThmCoolChrgStg_861.Default  OutDataTypeStr=Enum: enmThmCoolChrgStg_861
  Constant7 : Constant  Value=enmThmCoolChrgStg_861.Stg_Lv1Red  OutDataTypeStr=Enum: enmThmCoolChrgStg_861
  Constant8 : Constant  Value=enmThmCoolChrgStg_861.Stg_Lv1Res  OutDataTypeStr=Enum: enmThmCoolChrgStg_861
  Constant9 : Constant  Value=enmThmCoolChrgStg_861.Stg_Lv2Red  OutDataTypeStr=Enum: enmThmCoolChrgStg_861
  Data Type Conversion{3..8} (6 alike) : DataTypeConversion  OutDataTypeStr=uint8
  Relational Operator{,1..5} (6 alike) : RelationalOperator  Operator=~=  OutDataTypeStr=boolean  RndMeth=Simplest
  Switch{1..6} (6 alike) : Switch  Criteria=u2 ~= 0
  BTMR_pClntPwrReq : Outport  InitialOutput=0
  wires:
  BTMR_stsClntStg/1 -> Relational Operator5/1, Relational Operator4/1, Relational Operator3/1, Relational Operator1/1, Relational Operator/1, Relational Operator2/1
  Switch5/1 -> Switch4/1
  Relational Operator/1 -> Switch1/2
  Relational Operator3/1 -> Switch4/2
  Data Type Conversion6/1 -> Relational Operator3/2
  Constant9/1 -> Data Type Conversion6/1
  Switch2/1 -> Switch1/1
  Constant3/1 -> Switch1/3
  Constant10/1 -> Data Type Conversion7/1
  Relational Operator4/1 -> Switch5/2
  Switch6/1 -> Switch5/1
  Data Type Conversion3/1 -> Relational Operator/2
  Data Type Conversion7/1 -> Relational Operator4/2
  Constant6/1 -> Data Type Conversion3/1
  Switch1/1 -> BTMR_pClntPwrReq/1
  Constant13/1 -> Switch6/3
  Constant2/1 -> Switch6/1
  Constant4/1 -> Switch3/3
  Switch3/1 -> Switch2/1
  Constant5/1 -> Switch4/3
  Constant8/1 -> Data Type Conversion5/1
  Relational Operator2/1 -> Switch3/2
  Constant12/1 -> Switch5/3
  Data Type Conversion5/1 -> Relational Operator2/2
  Switch4/1 -> Switch3/1
  Data Type Conversion8/1 -> Relational Operator5/2
  Constant11/1 -> Data Type Conversion8/1
  Relational Operator5/1 -> Switch6/2
  Constant1/1 -> Switch2/3
  Relational Operator1/1 -> Switch2/2
  Data Type Conversion4/1 -> Relational Operator1/2
  Constant7/1 -> Data Type Conversion4/1

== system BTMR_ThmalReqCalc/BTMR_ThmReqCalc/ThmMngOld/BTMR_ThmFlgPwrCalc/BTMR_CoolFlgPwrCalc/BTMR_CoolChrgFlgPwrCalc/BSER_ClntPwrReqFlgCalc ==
  BTMR_stsClntStg : Inport
  Constant4 : Constant  Value=enmThmCoolFlg.COOL  OutDataTypeStr=Enum: enmThmCoolFlg
  Constant5 : Constant  Value=enmThmCoolFlg.INACTIVE  OutDataTypeStr=Enum: enmThmCoolFlg
  Constant6 : Constant  Value=enmThmCoolChrgStg_861.Default  OutDataTypeStr=Enum: enmThmCoolChrgStg_861
  Data Type Conversion1 : DataTypeConversion  OutDataTypeStr=uint8
  Data Type Conversion2 : DataTypeConversion  OutDataTypeStr=uint8
  Data Type Conversion3 : DataTypeConversion  OutDataTypeStr=uint8
  Relational Operator : RelationalOperator  Operator=~=  OutDataTypeStr=boolean  RndMeth=Simplest
  Switch : Switch  Criteria=u2 ~= 0
  BTMR_flgClntPwrReq : Outport  InitialOutput=0
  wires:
  Data Type Conversion2/1 -> Switch/3
  Data Type Conversion1/1 -> Switch/1
  Constant4/1 -> Data Type Conversion1/1
  Switch/1 -> BTMR_flgClntPwrReq/1
  Constant5/1 -> Data Type Conversion2/1
  Data Type Conversion3/1 -> Relational Operator/2
  Constant6/1 -> Data Type Conversion3/1
  Relational Operator/1 -> Switch/2
  BTMR_stsClntStg/1 -> Relational Operator/1

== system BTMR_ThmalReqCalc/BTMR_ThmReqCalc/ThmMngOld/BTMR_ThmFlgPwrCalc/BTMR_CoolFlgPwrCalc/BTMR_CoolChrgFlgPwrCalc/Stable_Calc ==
  source_Uint : Inport
  cntStable : Inport  Port=2
  Chart : Stateflow chart  TreatAsAtomicUnit=on
  Delay1 : Delay  DelayLength=1  InitialCondition=0
  Detect Change : simulink/Logic and Bit Operations/Detect Change  vinit=0  OutDataTypeStr=boolean
  Switch : Switch  Criteria=u2 ~= 0
  stableOut : Outport
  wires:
  source_Uint/1 -> Detect Change/1, Switch/3
  Switch/1 -> stableOut/1, Delay1/1
  Delay1/1 -> Switch/1
  Chart/1(flg_out) -> Switch/2
  cntStable/1 -> Chart/2(cntStable)
  Detect Change/1 -> Chart/1(trigger_in)

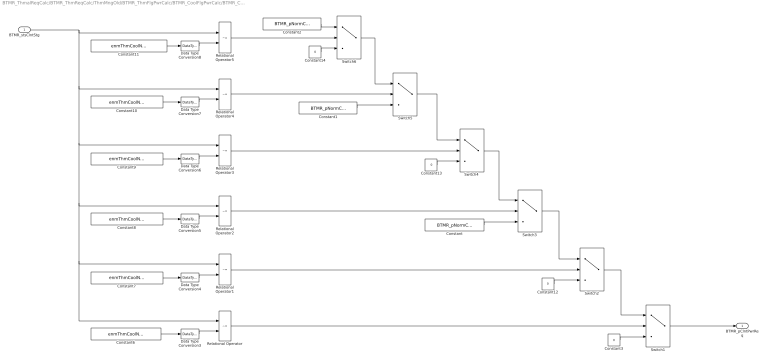
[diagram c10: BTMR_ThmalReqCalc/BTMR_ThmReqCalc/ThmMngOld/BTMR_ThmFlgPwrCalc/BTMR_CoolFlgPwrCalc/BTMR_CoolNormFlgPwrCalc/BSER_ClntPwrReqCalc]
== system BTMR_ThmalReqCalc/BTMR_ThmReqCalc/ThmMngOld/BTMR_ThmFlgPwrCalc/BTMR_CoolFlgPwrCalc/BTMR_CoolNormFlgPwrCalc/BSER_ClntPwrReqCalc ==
  BTMR_stsClntStg : Inport
  Constant : Constant  Value=BTMR_pNormClntPwrLv1_C
  Constant1 : Constant  Value=BTMR_pNormClntPwrLv2_C
  Constant10 : Constant  Value=enmThmCoolNormStg_861.Stg_Lv2Res  OutDataTypeStr=Enum: enmThmCoolNormStg_861
  Constant11 : Constant  Value=enmThmCoolNormStg_861.Stg_Lv3Red  OutDataTypeStr=Enum: enmThmCoolNormStg_861
  Constant{3,12..14} (4 alike) : Constant  Value=0  OutDataTypeStr=single
  Constant2 : Constant  Value=BTMR_pNormClntPwrLv3_C
  Constant6 : Constant  Value=enmThmCoolNormStg_861.Default  OutDataTypeStr=Enum: enmThmCoolNormStg_861
  Constant7 : Constant  Value=enmThmCoolNormStg_861.Stg_Lv1Red  OutDataTypeStr=Enum: enmThmCoolNormStg_861
  Constant8 : Constant  Value=enmThmCoolNormStg_861.Stg_Lv1Res  OutDataTypeStr=Enum: enmThmCoolNormStg_861
  Constant9 : Constant  Value=enmThmCoolNormStg_861.Stg_Lv2Red  OutDataTypeStr=Enum: enmThmCoolNormStg_861
  Data Type Conversion{3..8} (6 alike) : DataTypeConversion  OutDataTypeStr=uint8
  Relational Operator{,1..5} (6 alike) : RelationalOperator  Operator=~=  OutDataTypeStr=boolean  RndMeth=Simplest
  Switch{1..6} (6 alike) : Switch  Criteria=u2 ~= 0
  BTMR_pClntPwrReq : Outport  InitialOutput=0
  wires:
  BTMR_stsClntStg/1 -> Relational Operator5/1, Relational Operator4/1, Relational Operator3/1, Relational Operator1/1, Relational Operator/1, Relational Operator2/1
  Switch5/1 -> Switch4/1
  Relational Operator/1 -> Switch1/2
  Relational Operator3/1 -> Switch4/2
  Data Type Conversion6/1 -> Relational Operator3/2
  Constant9/1 -> Data Type Conversion6/1
  Switch2/1 -> Switch1/1
  Constant3/1 -> Switch1/3
  Constant10/1 -> Data Type Conversion7/1
  Relational Operator4/1 -> Switch5/2
  Switch6/1 -> Switch5/1
  Data Type Conversion3/1 -> Relational Operator/2
  Data Type Conversion7/1 -> Relational Operator4/2
  Constant6/1 -> Data Type Conversion3/1
  Switch1/1 -> BTMR_pClntPwrReq/1
  Constant14/1 -> Switch6/3
  Constant2/1 -> Switch6/1
  Constant/1 -> Switch3/3
  Switch3/1 -> Switch2/1
  Constant13/1 -> Switch4/3
  Constant8/1 -> Data Type Conversion5/1
  Relational Operator2/1 -> Switch3/2
  Constant1/1 -> Switch5/3
  Data Type Conversion5/1 -> Relational Operator2/2
  Switch4/1 -> Switch3/1
  Data Type Conversion8/1 -> Relational Operator5/2
  Constant11/1 -> Data Type Conversion8/1
  Relational Operator5/1 -> Switch6/2
  Constant12/1 -> Switch2/3
  Relational Operator1/1 -> Switch2/2
  Data Type Conversion4/1 -> Relational Operator1/2
  Constant7/1 -> Data Type Conversion4/1

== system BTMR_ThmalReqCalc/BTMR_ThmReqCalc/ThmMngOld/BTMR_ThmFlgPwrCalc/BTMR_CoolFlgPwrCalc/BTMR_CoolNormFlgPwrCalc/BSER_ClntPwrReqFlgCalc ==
  BTMR_stsClntStg : Inport
  Constant4 : Constant  Value=enmThmCoolFlg.COOL  OutDataTypeStr=Enum: enmThmCoolFlg
  Constant5 : Constant  Value=enmThmCoolFlg.INACTIVE  OutDataTypeStr=Enum: enmThmCoolFlg
  Constant6 : Constant  Value=enmThmCoolNormStg_861.Default  OutDataTypeStr=Enum: enmThmCoolNormStg_861
  Data Type Conversion1 : DataTypeConversion  OutDataTypeStr=uint8
  Data Type Conversion2 : DataTypeConversion  OutDataTypeStr=uint8
  Data Type Conversion3 : DataTypeConversion  OutDataTypeStr=uint8
  Relational Operator : RelationalOperator  Operator=~=  OutDataTypeStr=boolean  RndMeth=Simplest
  Switch : Switch  Criteria=u2 ~= 0
  BTMR_flgClntPwrReq : Outport  InitialOutput=0
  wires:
  Data Type Conversion2/1 -> Switch/3
  Data Type Conversion1/1 -> Switch/1
  Constant4/1 -> Data Type Conversion1/1
  Switch/1 -> BTMR_flgClntPwrReq/1
  Constant5/1 -> Data Type Conversion2/1
  Data Type Conversion3/1 -> Relational Operator/2
  Constant6/1 -> Data Type Conversion3/1
  BTMR_stsClntStg/1 -> Relational Operator/1
  Relational Operator/1 -> Switch/2

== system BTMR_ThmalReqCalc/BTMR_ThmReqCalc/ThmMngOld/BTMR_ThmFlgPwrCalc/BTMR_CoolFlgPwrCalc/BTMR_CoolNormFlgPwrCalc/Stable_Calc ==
  source_Uint : Inport
  cntStable : Inport  Port=2
  Chart : Stateflow chart  TreatAsAtomicUnit=on
  Delay1 : Delay  DelayLength=1  InitialCondition=0
  Detect Change : simulink/Logic and Bit Operations/Detect Change  vinit=0  OutDataTypeStr=boolean
  Switch : Switch  Criteria=u2 ~= 0
  stableOut : Outport
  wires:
  source_Uint/1 -> Detect Change/1, Switch/3
  Switch/1 -> stableOut/1, Delay1/1
  Delay1/1 -> Switch/1
  Chart/1(flg_out) -> Switch/2
  cntStable/1 -> Chart/2(cntStable)
  Detect Change/1 -> Chart/1(trigger_in)

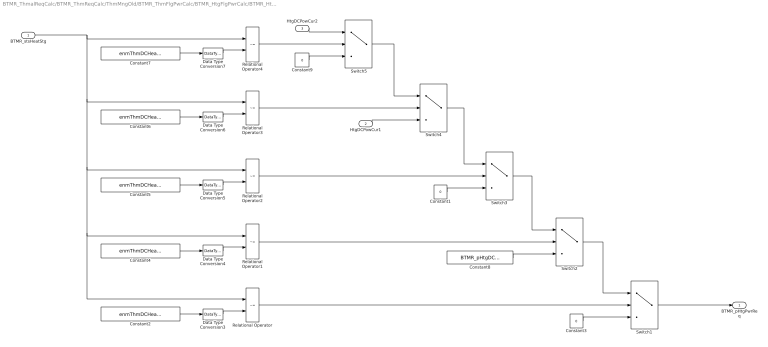
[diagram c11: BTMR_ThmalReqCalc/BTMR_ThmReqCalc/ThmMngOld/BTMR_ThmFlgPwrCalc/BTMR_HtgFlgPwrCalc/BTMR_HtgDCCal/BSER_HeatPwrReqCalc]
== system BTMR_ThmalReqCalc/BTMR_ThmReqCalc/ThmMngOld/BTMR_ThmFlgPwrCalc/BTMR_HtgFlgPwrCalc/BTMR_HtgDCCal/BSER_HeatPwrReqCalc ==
  BTMR_stsHeatStg : Inport
  HtgDCPowCur1 : Inport  Port=2
  HtgDCPowCur2 : Inport  Port=3
  Constant1 : Constant  Value=0  OutDataTypeStr=single
  Constant2 : Constant  Value=enmThmDCHeatStg_861.Default  OutDataTypeStr=Enum: enmThmDCHeatStg_861
  Constant3 : Constant  Value=0  OutDataTypeStr=single
  Constant4 : Constant  Value=enmThmDCHeatStg_861.Stg_Lv1  OutDataTypeStr=Enum: enmThmDCHeatStg_861
  Constant5 : Constant  Value=enmThmDCHeatStg_861.Stg_Lv2Red  OutDataTypeStr=Enum: enmThmDCHeatStg_861
  Constant6 : Constant  Value=enmThmDCHeatStg_861.Stg_Lv2Res  OutDataTypeStr=Enum: enmThmDCHeatStg_861
  Constant7 : Constant  Value=enmThmDCHeatStg_861.Stg_Lv3Red  OutDataTypeStr=Enum: enmThmDCHeatStg_861
  Constant8 : Constant  Value=BTMR_pHtgDCPwrReq_C
  Constant9 : Constant  Value=0  OutDataTypeStr=single
  Data Type Conversion{3..7} (5 alike) : DataTypeConversion  OutDataTypeStr=uint8
  Relational Operator{,1..4} (5 alike) : RelationalOperator  Operator=~=  OutDataTypeStr=boolean  RndMeth=Simplest
  Switch{1..5} (5 alike) : Switch  Criteria=u2 ~= 0
  BTMR_pHtgPwrReq : Outport  InitialOutput=0
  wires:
  BTMR_stsHeatStg/1 -> Relational Operator4/1, Relational Operator3/1, Relational Operator1/1, Relational Operator/1, Relational Operator2/1
  Switch5/1 -> Switch4/1
  Relational Operator/1 -> Switch1/2
  Relational Operator3/1 -> Switch4/2
  Data Type Conversion6/1 -> Relational Operator3/2
  Constant6/1 -> Data Type Conversion6/1
  Switch2/1 -> Switch1/1
  Constant3/1 -> Switch1/3
  Constant7/1 -> Data Type Conversion7/1
  Relational Operator4/1 -> Switch5/2
  Data Type Conversion3/1 -> Relational Operator/2
  Data Type Conversion7/1 -> Relational Operator4/2
  Constant2/1 -> Data Type Conversion3/1
  Switch1/1 -> BTMR_pHtgPwrReq/1
  Constant1/1 -> Switch3/3
  Switch3/1 -> Switch2/1
  HtgDCPowCur1/1 -> Switch4/3
  Constant5/1 -> Data Type Conversion5/1
  Relational Operator2/1 -> Switch3/2
  Constant9/1 -> Switch5/3
  Data Type Conversion5/1 -> Relational Operator2/2
  Switch4/1 -> Switch3/1
  Constant8/1 -> Switch2/3
  Relational Operator1/1 -> Switch2/2
  Data Type Conversion4/1 -> Relational Operator1/2
  Constant4/1 -> Data Type Conversion4/1
  HtgDCPowCur2/1 -> Switch5/1

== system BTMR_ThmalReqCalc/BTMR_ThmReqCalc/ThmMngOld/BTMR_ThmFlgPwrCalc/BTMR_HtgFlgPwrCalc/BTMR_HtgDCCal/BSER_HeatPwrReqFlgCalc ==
  BTMR_stsHeatStg : Inport
  Constant1 : Constant  Value=enmThmHeatFlg.ACTIVE  OutDataTypeStr=Enum: enmThmHeatFlg
  Constant5 : Constant  Value=enmThmHeatFlg.INACTIVE  OutDataTypeStr=Enum: enmThmHeatFlg
  Constant6 : Constant  Value=enmThmDCHeatStg_861.Default  OutDataTypeStr=Enum: enmThmDCHeatStg_861
  Data Type Conversion1 : DataTypeConversion  OutDataTypeStr=uint8
  Data Type Conversion2 : DataTypeConversion  OutDataTypeStr=uint8
  Data Type Conversion3 : DataTypeConversion  OutDataTypeStr=uint8
  Relational Operator : RelationalOperator  Operator=~=  OutDataTypeStr=boolean  RndMeth=Simplest
  Switch : Switch  Criteria=u2 ~= 0
  BTMR_flgHtgPwrReq : Outport  InitialOutput=0
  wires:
  Data Type Conversion2/1 -> Switch/3
  Data Type Conversion1/1 -> Switch/1
  Constant1/1 -> Data Type Conversion1/1
  Switch/1 -> BTMR_flgHtgPwrReq/1
  Constant5/1 -> Data Type Conversion2/1
  Data Type Conversion3/1 -> Relational Operator/2
  Constant6/1 -> Data Type Conversion3/1
  Relational Operator/1 -> Switch/2
  BTMR_stsHeatStg/1 -> Relational Operator/1

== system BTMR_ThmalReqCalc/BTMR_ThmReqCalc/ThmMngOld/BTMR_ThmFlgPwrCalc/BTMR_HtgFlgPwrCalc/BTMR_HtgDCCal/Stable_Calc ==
  source_Uint : Inport
  cntStable : Inport  Port=2
  Chart : Stateflow chart  TreatAsAtomicUnit=on
  Delay1 : Delay  DelayLength=1  InitialCondition=0
  Detect Change : simulink/Logic and Bit Operations/Detect Change  vinit=0  OutDataTypeStr=boolean
  Switch : Switch  Criteria=u2 ~= 0
  stableOut : Outport
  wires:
  source_Uint/1 -> Detect Change/1, Switch/3
  Switch/1 -> stableOut/1, Delay1/1
  Delay1/1 -> Switch/1
  Chart/1(flg_out) -> Switch/2
  cntStable/1 -> Chart/2(cntStable)
  Detect Change/1 -> Chart/1(trigger_in)

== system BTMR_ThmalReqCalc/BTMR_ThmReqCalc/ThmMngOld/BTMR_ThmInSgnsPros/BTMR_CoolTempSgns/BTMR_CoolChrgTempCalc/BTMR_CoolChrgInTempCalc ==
  BSPR_tCellTempMax : Inport
  BTMR_CoolChrgDnaTempCalc : Subsystem
  BTMR_CoolChrgStage2EnaTempCalc : Subsystem
  BTMR_CoolChrgStage2ExtTempCalc : Subsystem
  BTMR_CoolChrgStage3EnaTempCalc : Subsystem
  BTMR_CoolChrgStage3ExtTempCalc : Subsystem
  Bus Creator : BusCreator  Inputs=5
  BTMR_flgCoolChrgInTempSgns : Outport
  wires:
  BTMR_CoolChrgStage2EnaTempCalc/1(BTMR_flgCoolChrgStage2EnaTemp) -> Bus Creator/2  "BTMR_flgCoolChrgStage2EnaTemp"
  BTMR_CoolChrgStage3EnaTempCalc/1(BTMR_flgCoolChrgStage3EnaTemp) -> Bus Creator/3  "BTMR_flgCoolChrgStage3EnaTemp"
  BTMR_CoolChrgStage3ExtTempCalc/1(BTMR_flgCoolChrgStage3ExtTemp) -> Bus Creator/5  "BTMR_flgCoolChrgStage3ExtTemp"
  BTMR_CoolChrgStage2ExtTempCalc/1(BTMR_flgCoolChrgStage2ExtTemp) -> Bus Creator/4  "BTMR_flgCoolChrgStage2ExtTemp"
  BSPR_tCellTempMax/1 -> BTMR_CoolChrgStage3ExtTempCalc/1(BSPR_tCellTempMax), BTMR_CoolChrgStage2ExtTempCalc/1(BSPR_tCellTempMax), BTMR_CoolChrgDnaTempCalc/1(BSPR_tCellTempMax), BTMR_CoolChrgStage2EnaTempCalc/1(BSPR_tCellTempMax), BTMR_CoolChrgStage3EnaTempCalc/1(BSPR_tCellTempMax)
  BTMR_CoolChrgDnaTempCalc/1(BTMR_flgCoolChrgDnaTemp) -> Bus Creator/1  "BTMR_flgCoolChrgDnaTemp"
  Bus Creator/1 -> BTMR_flgCoolChrgInTempSgns/1  "BTMR_flgCoolChrgInTempSgns"

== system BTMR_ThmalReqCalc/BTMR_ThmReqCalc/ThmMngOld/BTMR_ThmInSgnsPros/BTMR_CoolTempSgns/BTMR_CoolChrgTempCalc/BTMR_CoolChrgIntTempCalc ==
  BSPR_tClntUsT : Inport
  BTMR_CoolChrgStage1PowRedTempCalc : Subsystem
  BTMR_CoolChrgStage1PowResTempCalc : Subsystem
  BTMR_CoolChrgStage2PowRedTempCalc : Subsystem
  BTMR_CoolChrgStage2PowResTempCalc : Subsystem
  BTMR_CoolChrgStage3PowRedTempCalc : Subsystem
  BTMR_CoolChrgStage3PowResTempCalc : Subsystem
  Bus Creator : BusCreator  Inputs=6
  BTMR_flgCoolChrgIntTempSgns : Outport
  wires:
  BTMR_CoolChrgStage1PowRedTempCalc/1(BTMR_flgCoolChrgStage1PowRedTemp) -> Bus Creator/1  "BTMR_flgCoolChrgStage1PowRedTemp"
  BTMR_CoolChrgStage1PowResTempCalc/1(BTMR_flgCoolChrgStage1PowResTemp) -> Bus Creator/2  "BTMR_flgCoolChrgStage1PowResTemp"
  BTMR_CoolChrgStage2PowRedTempCalc/1(BTMR_flgCoolChrgStage2PowRedTemp) -> Bus Creator/3  "BTMR_flgCoolChrgStage2PowRedTemp"
  BTMR_CoolChrgStage2PowResTempCalc/1(BTMR_flgCoolChrgStage2PowResTemp) -> Bus Creator/4  "BTMR_flgCoolChrgStage2PowResTemp"
  BTMR_CoolChrgStage3PowRedTempCalc/1(BTMR_flgCoolChrgStage3PowRedTemp) -> Bus Creator/5  "BTMR_flgCoolChrgStage3PowRedTemp"
  BTMR_CoolChrgStage3PowResTempCalc/1(BTMR_flgCoolChrgStage3PowResTemp) -> Bus Creator/6  "BTMR_flgCoolChrgStage3PowResTemp"
  BSPR_tClntUsT/1 -> BTMR_CoolChrgStage1PowRedTempCalc/1(BSPR_tClntUsT), BTMR_CoolChrgStage1PowResTempCalc/1(BSPR_tClntUsT), BTMR_CoolChrgStage2PowRedTempCalc/1(BSPR_tClntUsT), BTMR_CoolChrgStage3PowResTempCalc/1(BSPR_tClntUsT), BTMR_CoolChrgStage3PowRedTempCalc/1(BSPR_tClntUsT), BTMR_CoolChrgStage2PowResTempCalc/1(BSPR_tClntUsT)
  Bus Creator/1 -> BTMR_flgCoolChrgIntTempSgns/1  "BTMR_flgCoolChrgIntTempSgns"

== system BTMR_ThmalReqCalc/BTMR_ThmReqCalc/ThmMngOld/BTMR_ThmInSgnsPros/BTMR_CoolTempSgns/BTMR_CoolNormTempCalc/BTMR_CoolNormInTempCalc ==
  BSPR_tCellTempMax : Inport
  BTMR_CoolNormDnaTempCalc : Subsystem
  BTMR_CoolNormStage2EnaTempCalc : Subsystem
  BTMR_CoolNormStage2ExtTempCalc : Subsystem
  BTMR_CoolNormStage3EnaTempCalc : Subsystem
  BTMR_CoolNormStage3ExtTempCalc : Subsystem
  Bus Creator : BusCreator  Inputs=5
  BTMR_flgCoolNormInTempSgns : Outport
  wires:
  BTMR_CoolNormDnaTempCalc/1(BTMR_flgCoolNormDnaTemp) -> Bus Creator/1  "BTMR_flgCoolNormDnaTemp"
  BTMR_CoolNormStage2EnaTempCalc/1(BTMR_flgCoolNormStage2EnaTemp) -> Bus Creator/2  "BTMR_flgCoolNormStage2EnaTemp"
  BTMR_CoolNormStage3EnaTempCalc/1(BTMR_flgCoolNormStage3EnaTemp) -> Bus Creator/3  "BTMR_flgCoolNormStage3EnaTemp"
  BTMR_CoolNormStage3ExtTempCalc/1(BTMR_flgCoolNormStage3ExtTemp) -> Bus Creator/5  "BTMR_flgCoolNormStage3ExtTemp"
  BTMR_CoolNormStage2ExtTempCalc/1(BTMR_flgCoolNormStage2ExtTemp) -> Bus Creator/4  "BTMR_flgCoolNormStage2ExtTemp"
  BSPR_tCellTempMax/1 -> BTMR_CoolNormDnaTempCalc/1(BSPR_tCellTempMax), BTMR_CoolNormStage2EnaTempCalc/1(BSPR_tCellTempMax), BTMR_CoolNormStage3ExtTempCalc/1(BSPR_tCellTempMax), BTMR_CoolNormStage2ExtTempCalc/1(BSPR_tCellTempMax), BTMR_CoolNormStage3EnaTempCalc/1(BSPR_tCellTempMax)
  Bus Creator/1 -> BTMR_flgCoolNormInTempSgns/1  "BTMR_flgCoolNormInTempSgns"

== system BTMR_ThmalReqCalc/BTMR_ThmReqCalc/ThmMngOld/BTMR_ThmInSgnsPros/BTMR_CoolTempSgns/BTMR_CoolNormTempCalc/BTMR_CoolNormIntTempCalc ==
  BSPR_tClntUsT : Inport
  BTMR_CoolNormPowRedTempCalc : Subsystem
  BTMR_CoolNormPowResTempCalc : Subsystem
  Bus Creator1 : BusCreator  Inputs=2
  BTMR_flgCoolNormIntTempSgns : Outport
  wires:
  BSPR_tClntUsT/1 -> BTMR_CoolNormPowResTempCalc/1(BSPR_tClntUsT), BTMR_CoolNormPowRedTempCalc/1(BSPR_tClntUsT)
  Bus Creator1/1 -> BTMR_flgCoolNormIntTempSgns/1  "BTMR_flgCoolNormIntTempSgns"
  BTMR_CoolNormPowResTempCalc/1(BTMR_flgCoolNormPowResTemp) -> Bus Creator1/2  "BTMR_flgCoolNormPowResTemp"
  BTMR_CoolNormPowRedTempCalc/1(BTMR_flgCoolNormPowRedTemp) -> Bus Creator1/1  "BTMR_flgCoolNormPowRedTemp"
